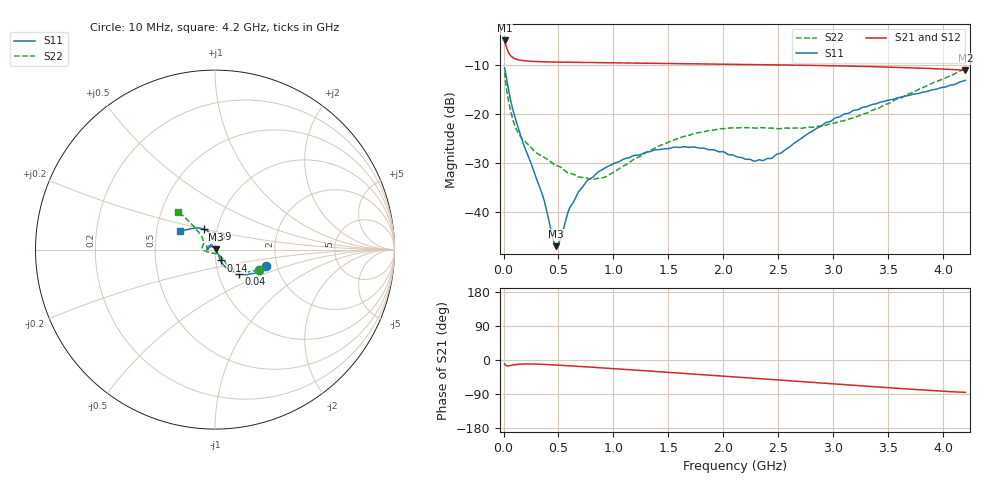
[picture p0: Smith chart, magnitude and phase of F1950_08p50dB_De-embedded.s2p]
! Integrated Device Technology
! Corporate Headquarters
! 6024 Silver Creek Valley Road
! San Jose, CA 95138  USA
! Phone:  1-408-284-8200
! Toll Free:  1-800-223-1366
! Webpage:  http://www.idt.com/
! Timing and RF Division
! 515 Groton Road, Suite 102
! Westford, MA 01886-6024
! Device:  F1950
! Description: 7-bit 0.25 dB Digital Step Attenuator
! Frequency:  150.0 -  4000.00 MHz
! Package:  4x4 mm Thin QFN Plastic Package: 24 pin
! Ports:  2 RF, 12 DC
!  Pin  1  = D0
!  Pin  2  = VDD
!  Pin  3  = Vmode
!  Pin  4  = GND
!  Pin  5  = RF1  =  Port 1
!  Pin  6  = GND
!  Pin  7  = GND
!  Pin  8  = GND
!  Pin  9  = GND
!  Pin 10  = GND
!  Pin 11  = GND
!  Pin 12  = GND
!  Pin 13  = GND
!  Pin 14  = RF2  =  Port 2
!  Pin 15  = GND
!  Pin 16  = LE
!  Pin 17  = CLK
!  Pin 18  = DATE
!  Pin 19  = D6
!  Pin 20  = D5
!  Pin 21  = D4
!  Pin 22  = D3
!  Pin 23  = D2
!  Pin 24  = D1
! State:  34
! Atten State:  8.50 dB
! Voltage:  +5.00 Volts
! Current:  Not Measured mA
! Data:  The device was measured on a the F195X evaluation board which has
!  individual transmission lines to the RF pins.  Data was collected
!  using a calibrated network analyzer.  The evaluation board was
!  de-embedded using a TRL calibration technique.
!  The reference plane is the edge of the package pin.
! Misc:  Board 2019
!  Action Tracker AT0250
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# GHz S dB R 50
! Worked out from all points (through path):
!   420 points, 10 MHz to 4.2 GHz, reference 50 ohm
!   highest |S21| = -4.90 dB at 10 MHz (marker M1); lowest = -11.0 dB at 4.2 GHz (marker M2)
!   group delay of S21, straight-line fit = 53.7 ps
!   lowest |S11| = -47.0 dB at 480 MHz (marker M3), VSWR 1.01, Z = 50.4 + j0.272 ohm
!   |S11| at or under -10 dB: start of sweep to end of sweep
!   |S22| runs from -33.4 to -10.6 dB; largest |S21 - S12| = 0.00043
!   S11 on the Smith chart (normalised r, x): 10 MHz: 1.75, -0.35; 40 MHz: 1.25, -0.35; 140 MHz: 1.06, -0.13; 3.39 GHz: 0.87, +0.20; 4.2 GHz: 0.66, +0.14
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0.01  -10.48 -18.0  -4.90 -10.5  -4.90 -10.5  -11.43 -25.3
0.04  -14.37 -45.4  -7.10 -15.6  -7.10 -15.6  -16.63 -47.5
0.09  -19.49 -60.3  -8.48 -13.1  -8.48 -13.1  -21.49 -50.6
0.14  -23.31 -62.6  -8.90 -11.2  -8.90 -11.2  -24.09 -50.3
0.35  -36.25 -43.9  -9.27 -11.4  -9.27 -11.4  -28.58 -54.1
0.45  -45.55 -0.8  -9.32 -12.8  -9.32 -12.8  -30.14 -57.6
0.48  -47.05 37.5  -9.33 -13.3  -9.33 -13.3  -30.51 -60.7
0.52  -45.44 79.5  -9.34 -13.9  -9.34 -13.9  -30.87 -62.5
0.6  -39.30 111.4  -9.37 -15.3  -9.37 -15.3  -32.12 -70.7
0.71  -35.16 125.6  -9.40 -17.3  -9.40 -17.3  -32.95 -84.5
0.92  -31.06 141.8  -9.46 -21.3  -9.46 -21.3  -32.91 -119.0
1.18  -28.51 157.5  -9.53 -26.3  -9.53 -26.3  -29.31 -151.5
1.41  -27.28 169.8  -9.59 -30.8  -9.59 -30.8  -26.54 -165.6
1.74  -26.75 179.5  -9.68 -37.4  -9.68 -37.4  -23.94 -177.8
2.11  -28.61 172.3  -9.79 -44.9  -9.78 -44.9  -22.82 172.1
2.28  -29.63 154.5  -9.84 -48.3  -9.83 -48.3  -22.84 167.6
2.43  -29.09 134.7  -9.88 -51.3  -9.88 -51.3  -22.86 163.4
2.81  -23.49 107.5  -10.01 -59.1  -10.01 -59.1  -22.69 149.3
3.1  -19.95 109.8  -10.13 -65.1  -10.13 -65.1  -21.32 140.8
3.39  -17.86 117.9  -10.29 -70.9  -10.28 -71.0  -18.93 135.1
3.51  -17.08 122.2  -10.36 -73.3  -10.35 -73.3  -17.75 133.4
4.2  -13.07 152.3  -11.02 -85.5  -11.01 -85.6  -10.65 133.9
